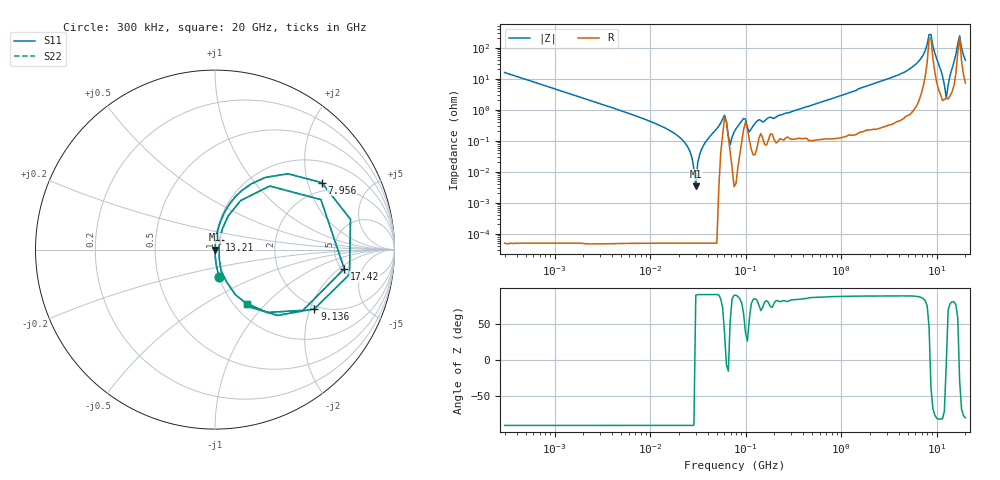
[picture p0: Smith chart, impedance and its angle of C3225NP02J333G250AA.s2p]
! S-Parameter Data Generated by TDK Corporation
! Copyright(C) 2025 TDK Corporation.
! All Rights Reserved.
! TDK P/N: C3225NP02J333G250AA (Multilayer Ceramic Chip Capacitor)
! Property: C=33nF
! Size(LxWxT): 3.2x2.5x2.5mm
! Model Type: s2p (Touchstone File Format Version 1.0)
! Frequency: DC=Yes Start=0.3MHz Stop=20000MHz 243points Log-sweep
! Model Generated on July 30, 2025
! Terms and conditions regarding TDK Simulation Models:
! 1)This simulation model is being provided solely for informational
!  purposes. Please refer to the specifications of the products in
!  terms of detailed characteristics of such products.
! 2)In no event shall TDK Corporation of any of its subsidiaries be
!  liable for any loss or damage arising, directly or indirectly,
!  from any information contained in this simulation model, including,
!  but not limited to loss or damages arising from any inaccuracies,
!  omissions or errors in connection with such information.
! 3)Any and all copyrights on this simulation model are owned by
!  TDK Corporation.  Duplication or redistribution of this simulation
!  model without prior written permission from TDK Corporation
!  is prohibited.
! 4)This simulation model is subject to any modification or change
!  without any prior notice.
! 5)Neither TDK Corporation nor any of its subsidiaries shall make any
!  warranty, express or implied, including but not limited to the
!  correctness, implied warranties of merchantability and fitness for
!  a particular purpose with respect to this simulation models.
! 6)The use of this simulation model shall be deemed to have consented
!  to the terms and conditions hereof.
! Port Assignments:
!  1 ---| |--- 2
! Applicable Conditions:
!  Temperature = 25 degC
!  DC Bias Voltage = 0 V
!  Small Signal Operation
# Hz S MA R 50
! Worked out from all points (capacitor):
!   242 points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, 300 kHz to 20 GHz, reference 50 ohm
!   read as one part in series: C = 33.4 nF near 314.2 kHz
!   lowest |Z| = 3.43 mohm at 30.11 MHz (marker M1)
!   series resonance near 29.82 MHz, so ESL is about 850 pH
!   S11 on the Smith chart (normalised r, x): 300 kHz: 1.00, -0.32; 7.956 GHz: 1.67, +2.46; 9.136 GHz: 1.89, -2.14; 13.21 GHz: 1.05, +0.12; 17.42 GHz: 5.24, -2.38; 20 GHz: 1.14, -0.78
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300000  0.1567 -81.0  0.9876 9.0  0.9876 9.0  0.1567 -81.0
1985118  0.02384 -88.7  0.9997 1.4  0.9997 1.4  0.02384 -88.7
1.254397e7  0.003164 -93.0  0.9998 0.2  0.9998 0.2  0.003164 -93.0
2.180869e7  0.001076 -99.4  0.9998 0.1  0.9998 0.1  0.001076 -99.4
3.011225e7  0.0001726 168.5  0.9998 -0.0  0.9998 -0.0  0.0001726 168.5
6.011549e7  0.006658 38.3  0.9948 -0.2  0.9948 -0.2  0.006658 38.3
6.902956e7  0.0007602 55.2  0.9996 -0.0  0.9996 -0.0  0.0007602 55.2
7.926541e7  0.002427 88.9  1 -0.1  1 -0.1  0.002427 88.9
9.531223e7  0.005253 63.6  0.9977 -0.3  0.9977 -0.3  0.005253 63.6
1.094453e8  0.001955 56.5  0.9989 -0.1  0.9989 -0.1  0.001955 56.5
5.008786e8  0.01431 85.1  0.9989 -0.8  0.9989 -0.8  0.01431 85.1
3.165055e9  0.101 82.4  0.9917 -5.8  0.9917 -5.8  0.101 82.4
6.318653e9  0.313 69.1  0.9353 -18.2  0.9353 -18.2  0.313 69.1
7.956199e9  0.7021 32.1  0.5496 -42.6  0.5496 -42.6  0.7021 32.1
8.72445e9  0.7618 -10.5  0.2842 28.0  0.2842 28.0  0.7618 -10.5
9.135962e9  0.6447 -30.8  0.5536 36.3  0.5536 36.3  0.6447 -30.8
1.150364e10  0.1224 -73.9  0.9733 6.9  0.9733 6.9  0.1224 -73.9
1.261444e10  0.02316 -6.0  0.977 0.1  0.977 0.1  0.02316 -6.0
1.320943e10  0.06163 65.8  0.9764 -3.3  0.9764 -3.3  0.06163 65.8
1.58836e10  0.4673 49.3  0.7775 -27.0  0.7775 -27.0  0.4673 49.3
1.741732e10  0.728 -8.4  0.299 20.6  0.299 20.6  0.728 -8.4
2e10  0.3492 -59.4  0.8757 20.1  0.8757 20.1  0.3492 -59.4
